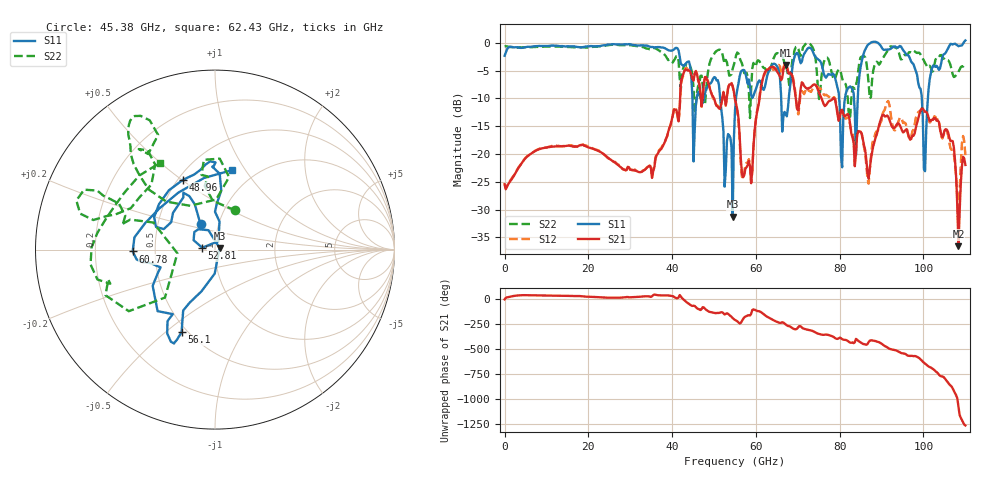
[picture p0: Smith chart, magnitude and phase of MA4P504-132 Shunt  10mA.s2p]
!Keysight Technologies,N5247B,US61255204,A.15.70.20
!Date: Friday, October 21, 2022 14:57:56
!Correction: S11(C  4-Port  )
!S31(C  4-Port  )
!S13(C  4-Port  )
!S33(C  4-Port  )
!S2P File: Measurements: S11, S31, S13, S33:
# Hz S  dB  R 50
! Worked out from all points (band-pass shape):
!   401 points, 10 MHz to 110 GHz, reference 50 ohm
!   highest |S21| = -3.96 dB at 67.1 GHz (marker M1); lowest = -36.6 dB at 108.4 GHz (marker M2)
!   |S21| within 3 dB of the highest: 42.14 GHz to 46.32 GHz (4.185 GHz wide, 9.46 % of centre); 61.5 GHz to 68.92 GHz (7.422 GHz wide, 11.4 % of centre)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
!   lowest |S11| = -31.3 dB at 54.46 GHz (marker M3), VSWR 1.06, Z = 52.6 + j1.01 ohm
!   |S11| at or under -10 dB: 51.48 GHz to 55.24 GHz (3.766 GHz wide, 7.06 % of centre); 66.03 GHz to 67.84 GHz (1.816 GHz wide, 2.71 % of centre); 79.86 GHz to 81.26 GHz (1.401 GHz wide, 1.74 % of centre)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
!   |S22| runs from -13.7 to 0.0 dB; largest |S21 - S12| = 0.24
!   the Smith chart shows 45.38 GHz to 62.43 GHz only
!   S11 on the Smith chart (normalised r, x): 45.38 GHz: 0.82, +0.24; 48.96 GHz: 0.53, +0.50; 52.81 GHz: 0.87, +0.02; 56.1 GHz: 0.46, -0.57; 60.78 GHz: 0.37, -0.01; 62.43 GHz: 0.78, +0.88
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1e7  -2.31 -179.5  -25.45 -8.3  -25.45 -8.0  -0.63 -179.8
1.843332e10  -0.79 117.8  -18.37 22.9  -18.39 23.0  -0.79 124.4
3.685665e10  -0.74 115.3  -19.54 32.2  -19.37 32.2  -1.35 122.1
4.373102e10  -3.38 16.9  -4.96 -44.8  -4.80 -42.7  -4.06 81.1
4.538088e10  -15.83 119.8  -5.61 -74.1  -5.54 -73.3  -12.18 62.4
4.895555e10  -7.38 114.7  -8.07 -133.3  -8.01 -131.6  -3.63 133.5
5.28052e10  -22.86 171.7  -11.15 -152.6  -11.33 -152.7  -3.06 127.2
5.445505e10  -31.29 20.6  -7.77 164.4  -7.86 163.6  -4.61 160.5
5.5005e10  -12.23 -108.0  -9.98 146.4  -10.22 144.6  -3.13 166.3
5.61049e10  -6.07 -112.0  -16.49 110.9  -17.37 114.6  -2.69 153.4
6.077948e10  -6.77 -178.7  -10.49 -127.3  -10.05 -122.7  -3.25 179.0
6.242932e10  -6.87 77.7  -4.92 -175.1  -5.16 -168.7  -4.85 122.2
6.71039e10  -12.79 -41.5  -3.96 101.2  -3.64 101.7  -4.32 45.5
7.342832e10  -1.30 138.7  -7.71 37.6  -8.41 35.9  -0.68 108.5
8.112762e10  -10.62 -29.0  -13.25 -51.7  -13.57 -52.6  -7.14 -125.4
8.525225e10  -3.32 38.9  -16.32 -86.3  -16.41 -84.8  -2.47 -23.3
9.185165e10  -1.16 90.9  -13.80 -140.5  -11.14 -134.6  -0.76 83.7
9.872602e10  -7.12 150.1  -13.69 131.5  -12.48 131.0  -1.76 176.9
1.003759e11  -23.10 -24.4  -12.38 69.6  -12.80 71.7  -3.62 -155.9
1.036756e11  -4.85 -33.8  -14.22 -39.8  -14.11 -36.4  -2.56 -89.8
1.083502e11  -0.59 22.3  -36.60 -3.8  -34.25 2.2  -5.17 -5.2
1.1e11  0.44 54.4  -21.97 172.0  -20.22 173.9  -4.08 16.6
